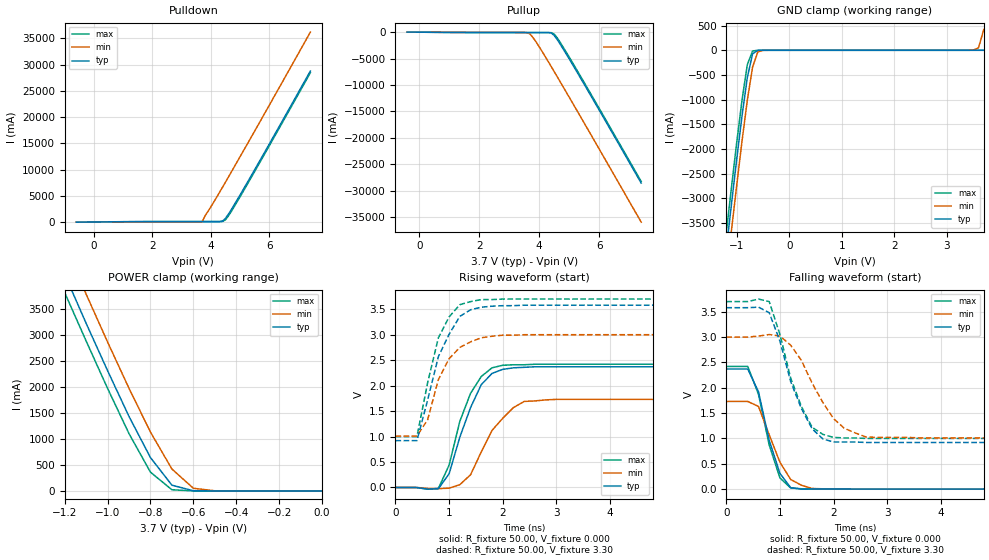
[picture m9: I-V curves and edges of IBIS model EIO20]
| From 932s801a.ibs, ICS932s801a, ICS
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|   Model EIO20
[Model]   EIO20
Model_type   I/O
Polarity   Non-Inverting
Enable   Active-High
Vinl =   0.80V
Vinh =   2.00V
C_comp   5.50pF   5.00pF   6.00pF
[Temperature Range]   27.00   70.00   0.000
[Voltage Range]   3.70V   3.00V   3.70V
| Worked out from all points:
|   slope of the pulldown table from 0 to 0.555 V, typ, clamps not added: 17.5 ohm
|   slope of the pullup table from 0 to 0.555 V, typ, clamps not added: 23.9 ohm
|   GND clamp passes 1 mA (typ) near -0.54 V on its own axis
|   POWER clamp passes 1 mA (typ) near -0.53 V on its own axis
|   rising waveform, R_fixture 50.00, V_fixture 0.000: 20-80 % time 488ps typ, 580ps min, 442ps max; typ from 0 V to 2.37 V
|   rising waveform, R_fixture 50.00, V_fixture 3.30: 20-80 % time 489ps typ, 446ps min, 405ps max; typ from 0.92 V to 3.58 V
|   falling waveform, R_fixture 50.00, V_fixture 0.000: 20-80 % time 345ps typ, 420ps min, 343ps max; typ from 2.37 V to 0 V
|   falling waveform, R_fixture 50.00, V_fixture 3.30: 20-80 % time 515ps typ, 630ps min, 478ps max; typ from 3.58 V to 0.92 V
[Pulldown]
| voltage   I(typ)   I(min)   I(max)
-600mV    -35.78mA   -28.06mA   -38.03mA
3.7V      73.16mA    49.6mA     76.55mA
3.8V      73.22mA    1.18A      76.61mA
4.4V      180mA      6.66A      99.51mA
4.5V      710mA      7.62A      440mA
4.6V      1.51A      8.59A      1.18A
5V        5.18A      12.48A     4.84A
5.6V      10.99A     18.37A     10.65A
7.4V      28.79A     36.22A     28.48A
[Pullup]
| voltage   I(typ)   I(min)   I(max)
-400mV    18.71mA    15.77mA    19.51mA
3.5V      -69.4mA    -47.13mA   -71.83mA
3.6V      -69.67mA   -78.48mA   -72.1mA
3.7V      -69.93mA   -380mA     -72.36mA
3.9V      -70.42mA   -1.88A     -72.83mA
4.4V      -140mA     -6.51A     -88.34mA
4.5V      -620mA     -7.47A     -370mA
4.6V      -1.39A     -8.43A     -1.07A
5.3V      -7.93A     -15.25A    -7.6A
7.4V      -28.59A    -36A       -28.29A
[GND_clamp]
| voltage   I(typ)   I(min)   I(max)
-3.7V     -28.52A    -29.01A    -28.21A
-1.2V     -4.03A     -4.56A     -3.69A
-1.1V     -3.1A      -3.63A     -2.76A
-1V       -2.19A     -2.72A     -1.85A
-900mV    -1.32A     -1.83A     -1A
-800mV    -550mA     -1.01A     -290mA
-700mV    -72.17mA   -340mA     -14.47mA
-600mV    -2.28mA    -32.47mA   -430uA
-500mV    -86.18uA   -1.3mA     -27.25uA
3.5V      67.02pA    2.14mA     61.7pA
3.6V      73.69pA    51.05mA    68.12pA
3.7V      80.4pA     420mA      74.55pA
[POWER_clamp]
| voltage   I(typ)   I(min)   I(max)
-3.7V     28.66A     29.18A     28.34A
-1.2V     4.16A      4.71A      3.81A
-1.1V     3.22A      3.78A      2.88A
-1V       2.31A      2.86A      1.97A
-900mV    1.43A      1.97A      1.1A
-800mV    640mA      1.13A      360mA
-700mV    110mA      420mA      22.36mA
-600mV    3.42mA     51.05mA    380uA
-500mV    80.59uA    2.14mA     6.04uA
0V        80.4pA     320pA      74.55pA
[Ramp]
| variable   typ   min   max
dV/dt_r   1.42/0.41n   1.04/0.57n   1.45/0.37n
dV/dt_f   1.58/0.45n   1.19/0.62n   1.62/0.40n
R_load = 50.00
[Rising Waveform]
R_fixture = 50.00
V_fixture = 0.000
V_fixture_min = 0.000
V_fixture_max = 0.000
| time   V(typ)   V(min)   V(max)
0s        140uV      81.39uV    150uV
800ps     -24.28mV   -22.29mV   -17.83mV
1ns       270mV      -13.26mV   440mV
1.2ns     990mV      55.93mV    1.3V
1.4ns     1.57V      250mV      1.85V
1.6ns     2.02V      700mV      2.18V
2ns       2.32V      1.36V      2.4V
2.4ns     2.36V      1.69V      2.41V
3ns       2.37V      1.73V      2.42V
10ns      2.37V      1.73V      2.42V
[Rising Waveform]
R_fixture = 50.00
V_fixture = 3.30
V_fixture_min = 3.00
V_fixture_max = 3.70
| time   V(typ)   V(min)   V(max)
0s        920mV      1.01V      1V
400ps     920mV      1.01V      1V
600ps     1.72V      1.33V      2.06V
800ps     2.57V      2.12V      2.94V
1ns       3.01V      2.53V      3.35V
1.2ns     3.36V      2.75V      3.59V
1.4ns     3.49V      2.86V      3.65V
1.8ns     3.56V      2.97V      3.69V
2.4ns     3.58V      3V         3.7V
10ns      3.58V      3V         3.7V
[Falling Waveform]
R_fixture = 50.00
V_fixture = 0.000
V_fixture_min = 0.000
V_fixture_max = 0.000
| time   V(typ)   V(min)   V(max)
0s        2.37V      1.73V      2.42V
400ps     2.37V      1.73V      2.42V
600ps     1.92V      1.63V      1.87V
800ps     960mV      1.07V      870mV
1ns       310mV      530mV      220mV
1.2ns     29.42mV    190mV      23.24mV
1.4ns     -1.13mV    76.14mV    6.83mV
1.6ns     3.07mV     12.36mV    3.11mV
1.8ns     2.53mV     5.98mV     2.06mV
10ns      140uV      84.11uV    140uV
[Falling Waveform]
R_fixture = 50.00
V_fixture = 3.30
V_fixture_min = 3.00
V_fixture_max = 3.70
| time   V(typ)   V(min)   V(max)
0s        3.58V      3V         3.7V
800ps     3.48V      3.05V      3.7V
1ns       2.92V      3.02V      3.05V
1.2ns     2.12V      2.84V      2.19V
1.4ns     1.59V      2.54V      1.63V
1.6ns     1.19V      2.09V      1.22V
2ns       930mV      1.39V      1.02V
2.2ns     930mV      1.2V       1.01V
2.8ns     920mV      1.02V      1V
10ns      920mV      1.01V      1V
